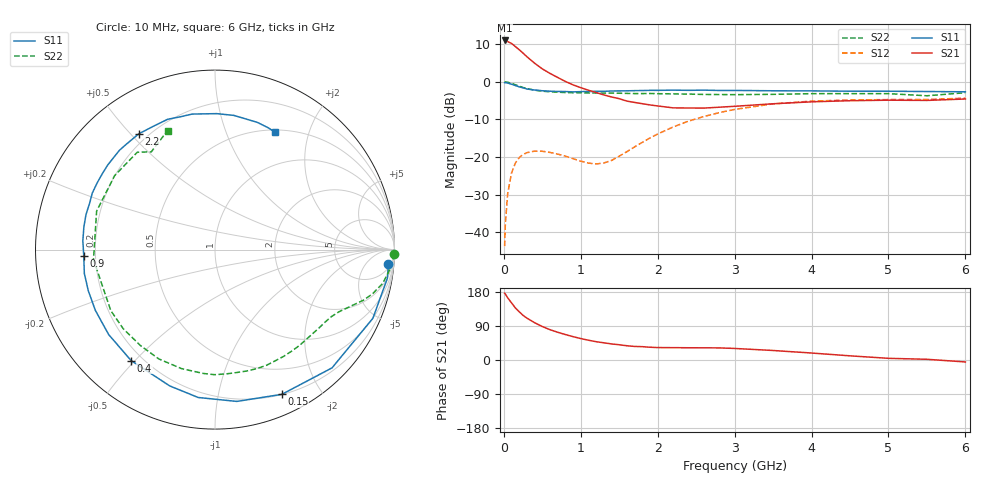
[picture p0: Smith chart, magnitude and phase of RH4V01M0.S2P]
! SIEMENS Small Signal Semiconductors
! BFR106
! Si NPN RF Bipolar Junction Transistor in SOT23
! VCE = 4 V  IC = 1 mA
! Common Emitter S-Parameters:  August  1996
# GHz  S  MA  R  50
!  f  S11  S21  S12  S22
! GHz  MAG  ANG  MAG  ANG  MAG  ANG  MAG  ANG
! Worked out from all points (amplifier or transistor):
!   36 points, 10 MHz to 6 GHz, reference 50 ohm
!   highest |S21| = 11.0 dB at 10 MHz (marker M1)
!   |S21| within 3 dB of that: start of sweep to 229.4 MHz
!   unconditionally stable (mu >= 1): 855.2 MHz to 2.045 GHz; 2.606 GHz to end of sweep
!   at 250 MHz: K = 0.27, MSG = 13.5 dB, |S12| = -19.3 dB
!   at 1.4 GHz: K = 1.44, MAG = 4.5 dB, |S12| = -20.9 dB
!   at 6 GHz: K = 1.02, MAG = -0.9 dB, |S12| = -4.4 dB
!   S11 on the Smith chart (normalised r, x): 10 MHz: 8, -21; 150 MHz: 0.20, -1.54; 400 MHz: 0.16, -0.49; 900 MHz: 0.15, -0.02; 2.2 GHz: 0.16, +0.53; 6 GHz: 0.53, +1.50
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0.01  0.9698 -4.7  3.537 176.3  0.0065 90.3  0.9999 -1.4
0.02  0.9735 -9.5  3.534 173.9  0.0131 85.5  0.996 -2.5
0.05  0.9593 -23.5  3.418 164.1  0.0326 77.3  0.9838 -6.0
0.1  0.927 -45.3  3.227 150.8  0.0612 65.4  0.9532 -11.4
0.15  0.8882 -65.2  2.933 137.4  0.0827 53.5  0.9112 -15.7
0.2  0.8546 -81.8  2.662 127.3  0.0979 45.6  0.8741 -18.8
0.25  0.8293 -96.5  2.399 117.7  0.1078 38.2  0.837 -21.3
0.3  0.8002 -108.4  2.149 110.5  0.1138 33.4  0.81 -23.4
0.4  0.775 -127.1  1.762 98.4  0.1193 25.1  0.772 -26.7
0.5  0.7583 -141.4  1.481 88.3  0.1189 19.9  0.7486 -29.9
0.6  0.7477 -153.1  1.289 80.0  0.1147 17.0  0.7347 -33.3
0.9  0.7321 -177.1  0.908 61.6  0.0948 18.4  0.7135 -44.4
1.1  0.7414 170.2  0.77 52.2  0.0828 29.3  0.7091 -52.8
1.3  0.7447 159.8  0.667 45.4  0.083 48.3  0.7046 -61.5
1.6  0.7567 146.3  0.552 37.6  0.1173 70.2  0.6991 -75.3
2.2  0.7724 123.4  0.449 32.6  0.2499 72.8  0.6888 -105.8
2.8  0.7646 104.5  0.458 31.9  0.3878 58.4  0.6751 -139.2
3.5  0.7576 89.3  0.509 25.1  0.5072 39.6  0.6793 -175.3
4.5  0.7476 76.1  0.559 11.0  0.5709 16.8  0.6947 143.6
5  0.7471 71.5  0.568 4.4  0.5785 8.4  0.6942 128.6
5.5  0.7404 66.2  0.564 1.9  0.5797 4.5  0.6501 123.1
6  0.7346 63.0  0.589 -5.2  0.6047 -3.4  0.714 111.7
